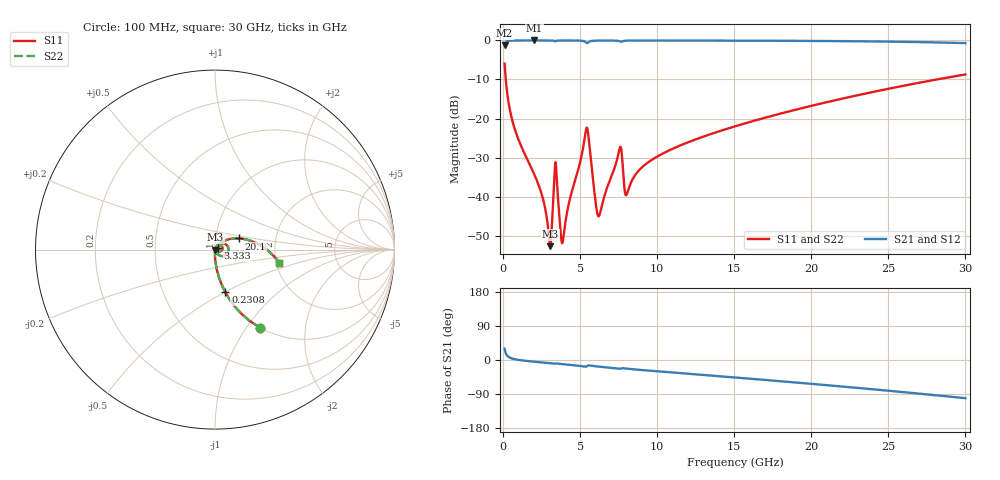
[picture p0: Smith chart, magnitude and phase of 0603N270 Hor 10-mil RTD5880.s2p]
# GHz S MA R 50
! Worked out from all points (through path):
!   3201 points, 100 MHz to 30 GHz, reference 50 ohm
!   highest |S21| = -0.01 dB at 2.025 GHz (marker M1); lowest = -1.3 dB at 100 MHz (marker M2)
!   group delay of S21, straight-line fit = 9.46 ps
!   lowest |S11| = -52.7 dB at 3.062 GHz (marker M3), VSWR 1.00, Z = 50.2 - j0.0752 ohm
!   |S11| at or under -10 dB: 175.1 MHz to 28.15 GHz (27.97 GHz wide, 198 % of centre)
!   |S22| runs from -52.7 to -5.9 dB; largest |S21 - S12| = 0
!   S11 on the Smith chart (normalised r, x): 100 MHz: 1.00, -1.17; 230.8 MHz: 1.00, -0.50; 3.333 GHz: 1.03, +0.02; 20.1 GHz: 1.29, +0.16; 30 GHz: 2.08, -0.36
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0.1  0.5048 -59.9  0.8629 30.0  0.8629 30.0  0.5048 -59.9
0.2308125  0.2448 -76.4  0.9692 13.5  0.9692 13.5  0.2448 -76.4
0.7634062  0.07301 -87.4  0.9966 2.0  0.9966 2.0  0.07301 -87.4
2.024812  0.01924 -90.9  0.9986 -4.6  0.9986 -4.6  0.01924 -90.9
2.56675  0.009737 -88.0  0.9984 -6.7  0.9984 -6.7  0.009737 -88.0
3.061969  0.002322 -18.8  0.9977 -8.6  0.9977 -8.6  0.002322 -18.8
3.332937  0.01789 30.2  0.9862 -10.0  0.9862 -10.0  0.01789 30.2
3.473094  0.01839 -54.3  0.9869 -9.0  0.9869 -9.0  0.01839 -54.3
3.725375  0.00367 -48.6  0.9971 -10.3  0.9971 -10.3  0.00367 -48.6
3.874875  0.002652 11.3  0.9975 -11.0  0.9975 -11.0  0.002652 11.3
5.089563  0.03303 56.6  0.9896 -16.1  0.9896 -16.1  0.03303 56.6
5.482  0.0725 -18.1  0.9275 -15.2  0.9275 -15.2  0.0725 -18.1
6.014594  0.008196 -45.1  0.9927 -16.7  0.9927 -16.7  0.008196 -45.1
6.210813  0.005615 1.5  0.9946 -17.5  0.9946 -17.5  0.005615 1.5
7.556312  0.04077 31.0  0.9754 -23.1  0.9754 -23.1  0.04077 31.0
8.0235  0.01066 25.2  0.9927 -22.9  0.9927 -22.9  0.01066 25.2
10.06978  0.03316 54.7  0.9962 -30.0  0.9962 -30.0  0.03316 54.7
15.05  0.07943 41.3  0.993 -46.1  0.993 -46.1  0.07943 41.3
20.03956  0.1459 25.3  0.9846 -63.0  0.9846 -63.0  0.1459 25.3
20.09562  0.1468 25.1  0.9845 -63.2  0.9845 -63.2  0.1468 25.1
25.01978  0.2408 7.6  0.9649 -81.1  0.9649 -81.1  0.2408 7.6
30  0.3663 -11.8  0.9238 -100.8  0.9238 -100.8  0.3663 -11.8
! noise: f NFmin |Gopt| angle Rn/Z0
0.1  0.0002944  0.9191  0.4013  0.0008035
3.417  0.014  0.9412  9.615  0.05284
6.743  0.007681  0.8045  18.89  0.007944
10.06  0.008225  0.7394  27.97  0.005959
13.39  0.009927  0.7189  36.89  0.006308
16.7  0.01181  0.7101  45.58  0.006853
20.03  0.01378  0.7065  54.06  0.007377
23.35  0.01585  0.7066  62.27  0.00786
26.67  0.01806  0.7096  70.25  0.008307
30  0.02046  0.7151  77.98  0.00872
